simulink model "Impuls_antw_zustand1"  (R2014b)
settings: Solver=ode45  StartTime=0.0  StopTime=10.0  MaxStep=0.1  RelTol=1e-3
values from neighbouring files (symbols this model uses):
  A = [-c1/m1, -k1/m1, c1/m1, k1/m1    [impuls_antw_zustand_1.m]    (also in modal_analyse_1.m; uebertragung_mechanik_1.m; uebertragung_zustand_1.m = [0,0,1/C1,-1/C1;0,-1/(C2*R2),0,1/C2;       -1/L1, 0 -Rg/L1, )
  B = [0, 0, 1/m2, 0]'    [impuls_antw_zustand_1.m]    (also in modal_analyse_1.m; uebertragung_mechanik_1.m; uebertragung_zustand_1.m = [0,0,1/L1,0]')
  C = [0 1 0 0;0 0 0 1]    [impuls_antw_zustand_1.m]    (also in impuls_antwort_1.m = 1e-07; impuls_antwort_2.m = 1e-07; impuls_antwort_3.m = 1e-07; impuls_antwort_4.m = 1e-07)

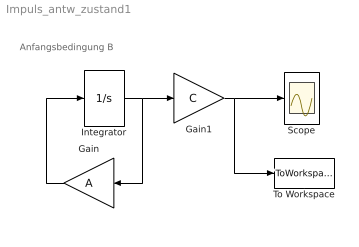
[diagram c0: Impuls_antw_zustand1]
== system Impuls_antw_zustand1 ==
  note: Anfangsbedingung B
  Gain : Gain  Gain=A  Multiplication=Matrix(K*u)  SampleTime=0
  Gain1 : Gain  Gain=C  Multiplication=Matrix(K*u)  SampleTime=0
  Integrator : Integrator  InitialCondition=B
  Scope : Scope
  To Workspace : ToWorkspace  VariableName=simout  SaveFormat=Timeseries  SampleTime=-1
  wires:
  Gain/1 -> Integrator/1
  Gain1/1 -> To Workspace/1, Scope/1
  Integrator/1 -> Gain1/1, Gain/1
